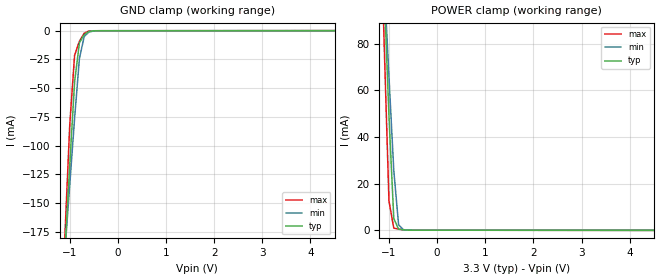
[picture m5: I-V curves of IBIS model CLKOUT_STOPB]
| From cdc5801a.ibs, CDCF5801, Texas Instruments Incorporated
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|   Clock Output  MODEL in STOPB state
[Model]   CLKOUT_STOPB
Model_type   Terminator
|Signals   CLKOUT,CLKOUTB
|variable   typ   min   max
C_comp   2.9pF   NA   NA
[Temperature Range] 25.0   0   85.0
[Voltage range]   3.3V   3.135V   3.465V
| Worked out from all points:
|   GND clamp passes 1 mA (typ) near -0.61 V on its own axis
|   POWER clamp passes 1 mA (typ) near -0.81 V on its own axis
[GND Clamp]
|   40C:3.3V:nominal   85C:3.0V:weak   0C:3.6V:strong
|   Voltage   I(typ)   I(min)   I(max)
-3.6V     -2.068A    -1.638A    -2.609A
-1.1V     -191.3mA   -191.5mA   -177.1mA
-1V       -116.5mA   -133.7mA   -81.41mA
-900mV    -44.6mA    -76.39mA   -21.41mA
-800mV    -10.47mA   -24.23mA   -9.133mA
-700mV    -3.389mA   -4.973mA   -2.14mA
-600mV    -608.7uA   -1.147mA   -204.2uA
-500mV    -67.94uA   -176.9uA   -28.97uA
-300mV    -4.228uA   -4.461uA   -5.896uA
6.6V      90.78uA    69.83uA    129.7uA
[POWER Clamp]
|   40C:3.3V:nominal   85C:3.0V:weak   0C:3.6V:strong
|   Voltage   I(typ)   I(min)   I(max)
-3.6V     1.449A     1.143A     1.831A
-1.2V     156.3mA    148.7mA    150.2mA
-1.1V     102.5mA    107.3mA    80.17mA
-1V       48.86mA    65.91mA    12.53mA
-900mV    5.055mA    25.69mA    889.8uA
-800mV    405.7uA    2.302mA    476.7uA
-700mV    149.3uA    208.8uA    222.2uA
6.6V      -83.54uA   -64.27uA   -119.4uA
